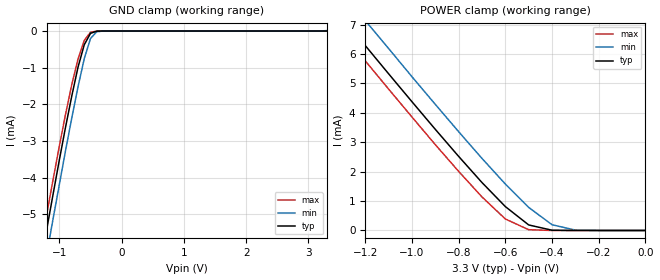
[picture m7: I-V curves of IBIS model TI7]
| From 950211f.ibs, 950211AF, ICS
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|   Model TI7
[Model]   TI7
Model_type   Input
Polarity   Non-Inverting
Vinl = 800.00mV
Vinh =   2.00V
C_comp   5.50pF   5.00pF   6.00pF
[Temperature Range]   27.00   70.00   0.00
[Voltage Range]   3.30V   3.00V   3.70V
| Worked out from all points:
|   GND clamp passes 1 mA (typ) near -0.70 V on its own axis
|   POWER clamp passes 1 mA (typ) near -0.62 V on its own axis
[GND_clamp]
| voltage   I(typ)   I(min)   I(max)
-3.3V     -25.98mA   -26.65mA   -25.56mA
-1.3V     -6.34mA    -7.02mA    -5.93mA
-1.2V     -5.39mA    -6.07mA    -4.98mA
-1.1V     -4.45mA    -5.12mA    -4.05mA
-900mV    -2.62mA    -3.26mA    -2.27mA
-800mV    -1.77mA    -2.37mA    -1.46mA
-700mV    -986.4uA   -1.52mA    -763.8uA
-600mV    -375.1uA   -753.1uA   -256.2uA
-500mV    -64.69uA   -205.5uA   -34.14uA
-400mV    -4.39uA    -20.4uA    -1.64uA
-300mV    -161.1nA   -1.12uA    -40.9nA
3.3V      123.3pA    12.3uA     91.17pA
[POWER_clamp]
| voltage   I(typ)   I(min)   I(max)
-3.3V     26.97mA    27.79mA    26.47mA
-1.4V     8.23mA     9.08mA     7.71mA
-1.3V     7.26mA     8.11mA     6.74mA
-1.2V     6.29mA     7.14mA     5.77mA
-1.1V     5.33mA     6.19mA     4.81mA
-800mV    2.52mA     3.36mA     2.01mA
-700mV    1.63mA     2.45mA     1.14mA
-600mV    812.4uA    1.58mA     391uA
-500mV    188.4uA    784.9uA    26.11uA
-400mV    7.94uA     195.1uA    419nA
-300mV    171.6nA    12.3uA     6.17nA
0V        123.3pA    259.4pA    135.8pA
